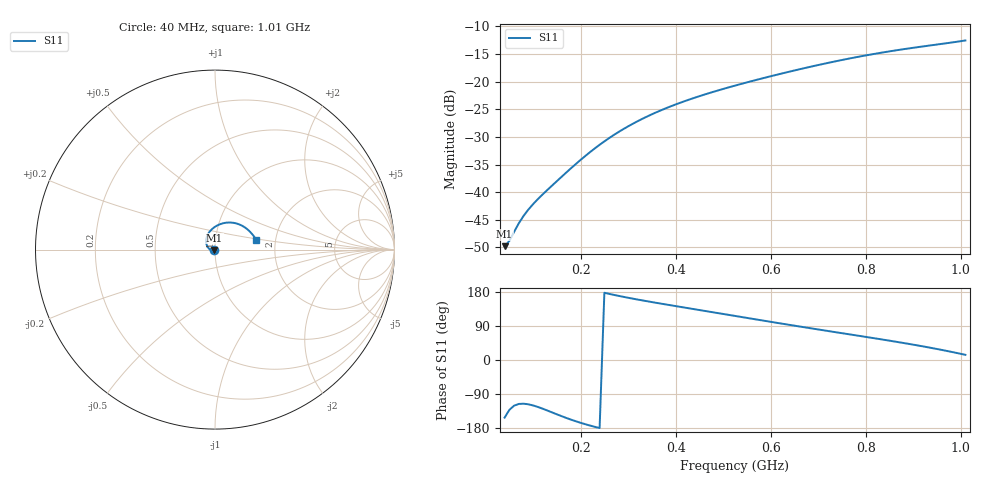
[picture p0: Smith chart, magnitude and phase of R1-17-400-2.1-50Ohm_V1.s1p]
!version-1
!date-08.2020
!Series
#	GHZ S RI R 50.0
!	FREQ.GHZ	S11RE	S11IM
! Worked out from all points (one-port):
!   98 points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, 40 MHz to 1.01 GHz, reference 50 ohm
!   lowest |S11| = -49.8 dB at 40 MHz (marker M1), VSWR 1.01, Z = 49.7 - j0.151 ohm
!   |S11| at or under -10 dB: start of sweep to end of sweep
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0.04  -0.00287 -0.00152
0.05  -0.00241 -0.00271
0.07  -0.0023 -0.00471
0.08  -0.00261 -0.00552
0.09  -0.00315 -0.00621
0.1  -0.00389 -0.00676
0.12  -0.00593 -0.00747
0.17  -0.0134 -0.00685
0.2  -0.019 -0.00483
0.23  -0.0249 -0.00156
0.26  -0.0307 0.00292
0.29  -0.0362 0.00856
0.32  -0.0411 0.0153
0.35  -0.0451 0.0231
0.38  -0.0479 0.0318
0.41  -0.0495 0.0413
0.46  -0.0488 0.0585
0.53  -0.0398 0.0843
0.59  -0.0242 0.1063
0.65  -0.00134 0.1261
0.71  0.0284 0.1415
0.77  0.064 0.15
0.83  0.104 0.1489
0.89  0.1465 0.1351
0.92  0.168 0.1224
0.95  0.1892 0.1052
0.98  0.2096 0.0831
1.01  0.229 0.0555
